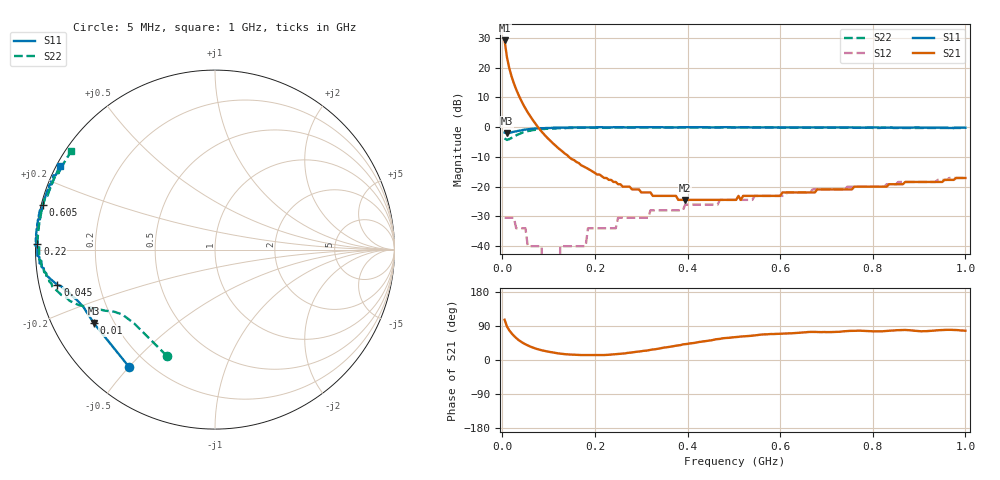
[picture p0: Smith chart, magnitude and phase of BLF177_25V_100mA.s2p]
! Filename:  BLF177_25V_100mA.s2p
! Philips part #: BLF177  !date: 21-05-2003
!Vdd=25V ; Idq=100mA
!D:\Vee measurements\measurement data\VDMOST\BLF177\25V_100mA_#1
# HZ S MA R 50
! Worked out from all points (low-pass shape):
!   200 points, 5 MHz to 1 GHz, reference 50 ohm
!   highest |S21| = 29.15 dB at 5 MHz (marker M1); lowest = -24.4 dB at 395 MHz (marker M2)
!   |S21| within 3 dB of the highest: start of sweep to 7.675 MHz
!   lowest |S11| = -2.0 dB at 10 MHz (marker M3), VSWR 8.52, Z = 6.31 - j13.7 ohm
!   |S11| at or under -10 dB: nowhere
!   |S22| runs from -4.3 to -0.1 dB; largest |S21 - S12| = 29
!   S11 on the Smith chart (normalised r, x): 5 MHz: 0.13, -0.50; 10 MHz: 0.13, -0.27; 45 MHz: 0.05, -0.11; 220 MHz: 0.01, +0.02; 605 MHz: 0.01, +0.13; 1 GHz: 0.01, +0.25
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5000000  0.81 -126.3  28.68 106.2  0.03 17.0  0.65 -114.4
1e7  0.79 -148.9  15.04 88.7  0.03 0.3  0.61 -137.6
1.5e7  0.8 -156.5  9.87 78.4  0.03 -8.8  0.63 -144.9
2e7  0.82 -160.1  7.13 70.5  0.03 -15.7  0.66 -148.4
2.5e7  0.84 -162.3  5.46 63.9  0.03 -21.3  0.7 -150.9
3e7  0.85 -164.0  4.32 58.0  0.02 -26.1  0.73 -153.0
4.5e7  0.9 -167.4  2.42 44.8  0.02 -35.3  0.82 -157.9
6e7  0.93 -169.8  1.54 35.7  0.01 -38.8  0.87 -162.1
8.5e7  0.96 -173.3  0.84 25.7  0.01 -27.2  0.93 -167.3
9e7  0.96 -173.8  0.76 24.3  0 -19.4  0.93 -168.2
1.2e8  0.98 -176.4  0.45 17.6  0 62.3  0.96 -172.5
1.25e8  0.98 -176.7  0.42 16.8  0.01 68.7  0.96 -173.0
1.75e8  0.99 -179.9  0.22 13.1  0.01 87.3  0.98 -177.5
1.85e8  0.99 179.7  0.2 13.0  0.02 88.0  0.98 -178.3
2.2e8  0.99 178.1  0.14 13.1  0.02 88.5  0.98 179.4
3.4e8  1 173.7  0.07 30.5  0.04 87.4  0.99 173.2
3.95e8  1 171.9  0.06 41.9  0.05 87.4  0.99 170.7
5.05e8  0.99 168.4  0.06 60.6  0.06 85.7  0.99 166.0
6.05e8  0.99 165.3  0.08 69.8  0.07 84.3  0.98 162.0
6.7e8  0.99 163.1  0.08 74.1  0.09 84.1  0.98 159.3
8.35e8  0.98 157.7  0.11 77.0  0.11 84.2  0.98 152.6
1e9  0.98 151.7  0.14 77.3  0.14 79.6  0.97 145.6
